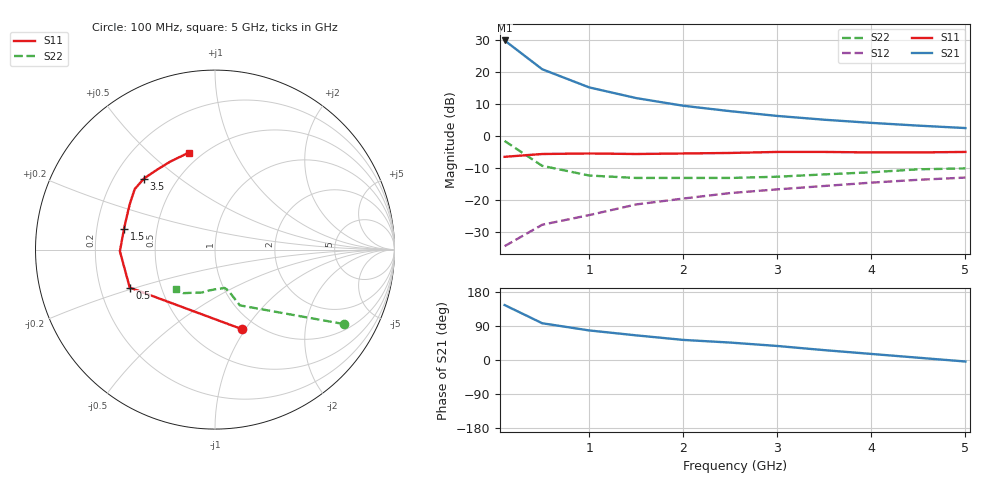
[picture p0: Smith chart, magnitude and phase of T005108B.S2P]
!AT-00510
!S-PARAMETERS at Vce=8V  Ic=20mA.  LAST UPDATED 07-21-92
!OBSOLETED Feb 1994 - nearest replacement: AT-41410
# ghz s ma r 50
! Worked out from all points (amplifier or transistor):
!   11 points, 100 MHz to 5 GHz, reference 50 ohm
!   highest |S21| = 29.7 dB at 100 MHz (marker M1)
!   |S21| within 3 dB of that: start of sweep to 233.6 MHz
!   unconditionally stable (mu >= 1): 873.1 MHz to end of sweep
!   at 500 MHz: K = 0.77, MSG = 24.2 dB, |S12| = -27.7 dB
!   at 2.5 GHz: K = 1.14, MAG = 10.5 dB, |S12| = -17.9 dB
!   at 5 GHz: K = 1.09, MAG = 5.9 dB, |S12| = -13.0 dB
!   S11 on the Smith chart (normalised r, x): 100 MHz: 0.85, -0.97; 500 MHz: 0.33, -0.19; 1.5 GHz: 0.32, +0.10; 3.5 GHz: 0.33, +0.38; 5 GHz: 0.43, +0.67
0.1  0.47 -71.0  30.66 145.0  0.019 63.0  0.83 -30.0
0.5  0.52 -156.0  10.9 97.0  0.041 51.0  0.34 -66.0
1  0.53 -179.0  5.68 78.0  0.058 52.0  0.24 -72.0
1.5  0.52 167.0  3.87 65.0  0.085 55.0  0.22 -76.0
2  0.53 156.0  2.94 53.0  0.105 51.0  0.22 -84.0
2.5  0.54 151.0  2.42 46.0  0.128 51.0  0.22 -88.0
3  0.56 143.0  2.04 37.0  0.146 50.0  0.23 -98.0
3.5  0.56 135.0  1.78 26.0  0.165 44.0  0.25 -107.0
4  0.55 126.0  1.59 16.0  0.186 39.0  0.27 -117.0
4.5  0.55 117.0  1.44 6.0  0.206 32.0  0.3 -126.0
5  0.56 105.0  1.32 -4.0  0.223 26.0  0.31 -135.0
